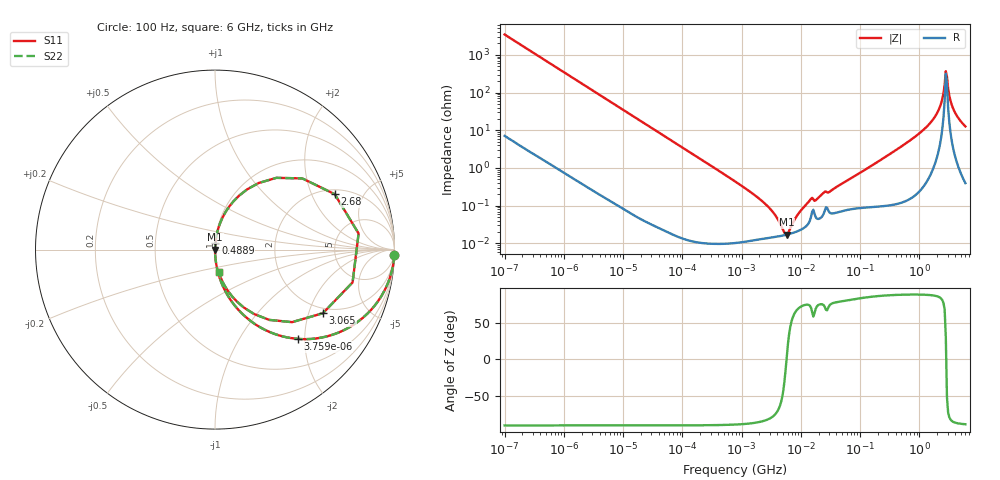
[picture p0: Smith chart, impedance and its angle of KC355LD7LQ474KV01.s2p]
!Murata Part Number: KC355LD7LQ474KV01
!These Parameters are Measured in Series Mode Connection
!Data Generated on Jun 19, 2026
!  o--ll--o
!Port1  Port2
!  o------o
!Operation Temp=25[degC], DC Bias Voltage=0[V]
!Freq. Start=100[Hz] Stop=6[GHz] 401[Steps]
# Hz S RI R 50
!Freq.(Hz) S11(Real) S11(Imag) S21(Real) S21(Imag) S12(Real) S12(Imag) S22(Real) S22(Imag)
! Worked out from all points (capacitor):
!   401 points, 100 Hz to 6 GHz, reference 50 ohm
!   read as one part in series: C = 458 nF near 109 Hz
!   lowest |Z| = 17.2 mohm at 5.809 MHz (marker M1)
!   series resonance near 5.735 MHz, so ESL is about 1.7 nH
!   S11 on the Smith chart (normalised r, x): 100 Hz: 1, -69; 3.759 kHz: 1.00, -1.85; 488.9 MHz: 1.00, +0.07; 2.68 GHz: 2.23, +2.99; 3.065 GHz: 1.80, -2.49; 6 GHz: 1.01, -0.25
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100  0.9991 -0.0288  0.00089 0.0288  0.00089 0.0288  0.9991 -0.0288
750  0.9552 -0.2059  0.0448 0.2059  0.0448 0.2059  0.9552 -0.2059
2008  0.7499 -0.432  0.2501 0.432  0.2501 0.432  0.7499 -0.432
3759  0.4624 -0.4975  0.5376 0.4975  0.5376 0.4975  0.4624 -0.4975
10066  0.1079 -0.3091  0.8921 0.3091  0.8921 0.3091  0.1079 -0.3091
40335  0.00771 -0.086  0.9923 0.086  0.9923 0.086  0.00771 -0.086
774597  0.000122 -0.00442  0.9999 0.00442  0.9999 0.00442  0.000122 -0.00442
2713602  0.000139 -0.000984  0.9999 0.000984  0.9999 0.000984  0.000139 -0.000984
5809218  0.000171 1.56e-05  0.9998 -1.56e-05  0.9998 -1.56e-05  0.000171 1.56e-05
9506416  0.000222 0.000633  0.9998 -0.000633  0.9998 -0.000633  0.000222 0.000633
1.555665e7  0.000701 0.00145  0.9993 -0.00145  0.9993 -0.00145  0.000701 0.00145
3.124326e8  0.00154 0.0229  0.9985 -0.0229  0.9985 -0.0229  0.00154 0.0229
4.888888e8  0.00251 0.0364  0.9975 -0.0364  0.9975 -0.0364  0.00251 0.0364
1.144649e9  0.0126 0.0974  0.9874 -0.0974  0.9874 -0.0974  0.0126 0.0974
1.873145e9  0.066 0.2207  0.934 -0.2207  0.934 -0.2207  0.066 0.2207
2.240541e9  0.1781 0.335  0.8219 -0.335  0.8219 -0.335  0.1781 0.335
2.450438e9  0.3422 0.3998  0.6578 -0.3998  0.6578 -0.3998  0.3422 0.3998
2.679998e9  0.6669 0.309  0.3331 -0.309  0.3331 -0.309  0.6669 0.309
3.065283e9  0.6012 -0.3544  0.3988 0.3544  0.3988 0.3544  0.6012 -0.3544
3.352442e9  0.3024 -0.3917  0.6976 0.3917  0.6976 0.3917  0.3024 -0.3917
3.8344e9  0.1221 -0.2895  0.8779 0.2895  0.8779 0.2895  0.1221 -0.2895
6e9  0.0195 -0.1235  0.9805 0.1235  0.9805 0.1235  0.0195 -0.1235
